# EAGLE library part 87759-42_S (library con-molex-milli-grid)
HEADER
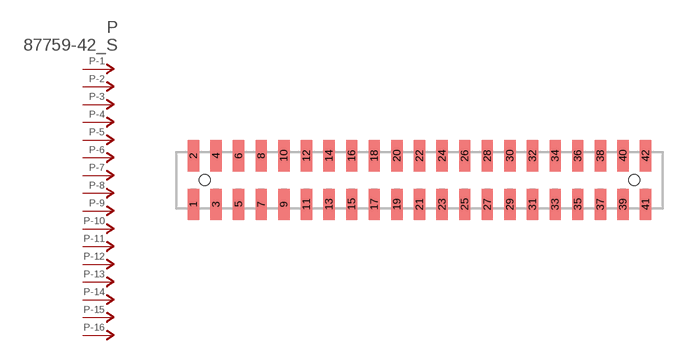
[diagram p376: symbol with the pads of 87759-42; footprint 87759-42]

Designator prefix P; gates -1=P-NV -2=P-N -3=P-N -4=P-N -5=P-N -6=P-N -7=P-N -8=P-N -9=P-N -10=P-N -11=P-N -12=P-N -13=P-N -14=P-N -15=P-N -16=P-N -17=P-N -18=P-N -19=P-N -20=P-N -21=P-N -22=P-N -23=P-N -24=P-N -25=P-N -26=P-N -27=P-N -28=P-N -29=P-N -30=P-N -31=P-N -32=P-N -33=P-N -34=P-N -35=P-N -36=P-N -37=P-N -38=P-N -39=P-N -40=P-N -41=P-N -42=P-N

## 87759-42_S  [87759-42]
1  -1:P  pas
2  -2:P  pas
3  -3:P  pas
4  -4:P  pas
5  -5:P  pas
6  -6:P  pas
7  -7:P  pas
8  -8:P  pas
9  -9:P  pas
10  -10:P  pas
11  -11:P  pas
12  -12:P  pas
13  -13:P  pas
14  -14:P  pas
15  -15:P  pas
16  -16:P  pas
17  -17:P  pas
18  -18:P  pas
19  -19:P  pas
20  -20:P  pas
21  -21:P  pas
22  -22:P  pas
23  -23:P  pas
24  -24:P  pas
25  -25:P  pas
26  -26:P  pas
27  -27:P  pas
28  -28:P  pas
29  -29:P  pas
30  -30:P  pas
31  -31:P  pas
32  -32:P  pas
33  -33:P  pas
34  -34:P  pas
35  -35:P  pas
36  -36:P  pas
37  -37:P  pas
38  -38:P  pas
39  -39:P  pas
40  -40:P  pas
41  -41:P  pas
42  -42:P  pas

## Footprint 87759-42 (pad centres in mm)
HEADER SMD Dual Row, Vertical
smd 1 x 2.75: 1 -20,-2.15; 2 -20,2.15; 3 -18,-2.15; 4 -18,2.15; 5 -16,-2.15; 6 -16,2.15; 7 -14,-2.15; 8 -14,2.15; 9 -12,-2.15; 10 -12,2.15; 11 -10,-2.15; 12 -10,2.15; 13 -8,-2.15; 14 -8,2.15; 15 -6,-2.15; 16 -6,2.15; 17 -4,-2.15; 18 -4,2.15; 19 -2,-2.15; 20 -2,2.15; 21 0,-2.15; 22 0,2.15; 23 2,-2.15; 24 2,2.15; 25 4,-2.15; 26 4,2.15; 27 6,-2.15; 28 6,2.15; 29 8,-2.15; 30 8,2.15; 31 10,-2.15; 32 10,2.15; 33 12,-2.15; 34 12,2.15; 35 14,-2.15; 36 14,2.15; 37 16,-2.15; 38 16,2.15; 39 18,-2.15; 40 18,2.15; 41 20,-2.15; 42 20,2.15
hole 1 at -19,0
hole 1 at 19,0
